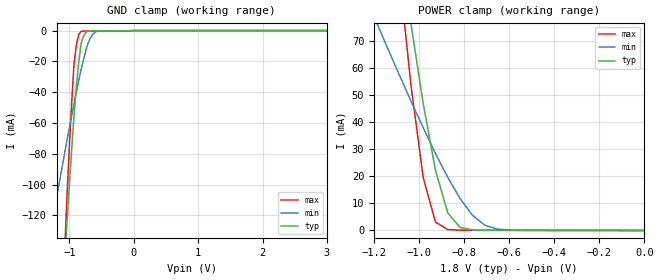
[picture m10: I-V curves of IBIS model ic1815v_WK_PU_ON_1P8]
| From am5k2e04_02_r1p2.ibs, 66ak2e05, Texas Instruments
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|   Model Cell ic1815v_WK_PU_ON_1P8
|WK_PU_ON_1P8
[Model]   ic1815v_WK_PU_ON_1P8
Model_type   Input
Polarity   Non-Inverting
Vinl =  0.63
Vinh =  1.17
C_comp   0.751145p   0.686962p   0.76914p
[Model Spec]
Vinl   0.63   0.567   0.693
Vinh   1.17   1.053   1.287
[Temperature Range]   25   125   -40
[Voltage Range]   1.8   1.62   1.98
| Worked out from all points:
|   GND clamp passes 1 mA (typ) near -0.74 V on its own axis
|   POWER clamp passes 1 mA (typ) near -0.81 V on its own axis
[POWER_clamp]
|   voltage   I(typ)   I(min)   I(max)
-1.8V     581.9mA    200.6mA    781mA
-1.182V   165.8mA    75.71mA    178.3mA
-1.073V   98.21mA    54.81mA    83.06mA
-1.055V   87.46mA    51.4mA     68.55mA
-1.036V   76.7mA     47.99mA    54.05mA
-981.8mV  47.07mA    38.07mA    19.62mA
-927.3mV  22.26mA    28.55mA    3.124mA
-872.7mV  6.543mA    19.68mA    337.6uA
-818.2mV  1.147mA    11.82mA    100.5uA
-763.6mV  196uA      5.683mA    78.63uA
-654.5mV  44.88uA    530.5uA    66.44uA
0V        41.88pA    124.8pA    49.32pA
[GND_clamp]
|   voltage   I(typ)   I(min)   I(max)
-1.8V     -691.6mA   -252.4mA   -924.6mA
-1.291V   -306.2mA   -129.9mA   -367.3mA
-1.073V   -148.9mA   -79.31mA   -141.7mA
-1.036V   -123.8mA   -71.08mA   -106.6mA
-1V       -99.8mA    -63.02mA   -74.62mA
-927.3mV  -54.59mA   -47.21mA   -20.98mA
-890.9mV  -35.89mA   -39.66mA   -9.288mA
-818.2mV  -8.233mA   -25.26mA   -525.7uA
-745.5mV  -1.184mA   -13.16mA   -261.9uA
-672.7mV  -234.1uA   -4.724mA   -243.2uA
-527.3mV  -140.9uA   -227.1uA   -231.4uA
3.6V      0A         0A         0A
